FUNCTION_BLOCK "Main"
VERSION : 0.1
   VAR_INPUT
      in1 : DInt;
      in2 : DInt;
   END_VAR

   VAR_OUTPUT
      out1 : DInt;
   END_VAR

   VAR_TEMP
      compResult : Bool;
   END_VAR

BEGIN
NETWORK
TITLE =
      L #in1;
      L #in2;
      -D;
      T #out1;
      L DINT#3000;
      <>D;
      = #compResult;
      CALL "__CPROVER_assert"
      (  condition                   := #compResult
      );
END_FUNCTION_BLOCK

